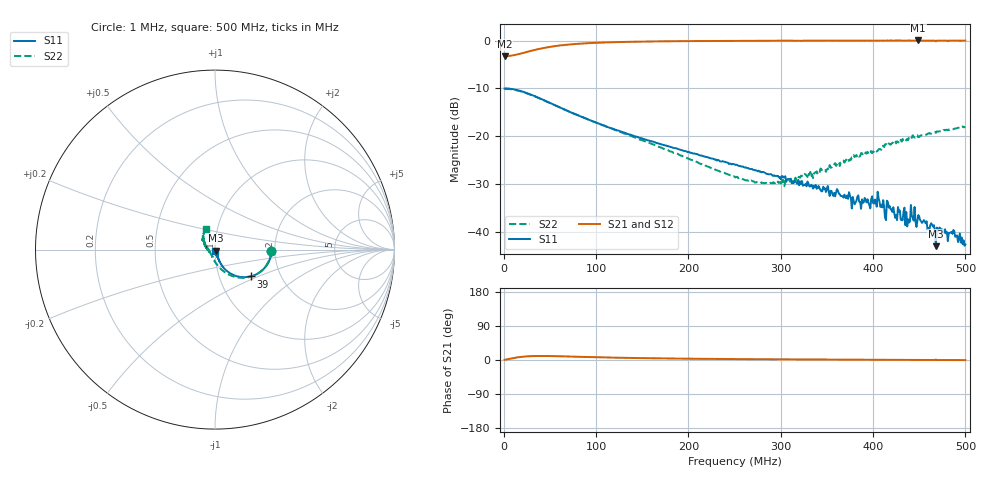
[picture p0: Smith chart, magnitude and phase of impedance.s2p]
# Hz S RI R 50.0
! written by SimSmith version 18.3b
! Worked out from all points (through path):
!   500 points, 1 MHz to 500 MHz, reference 50 ohm
!   highest |S21| = 0.01 dB at 449 MHz (marker M1); lowest = -3.3 dB at 1 MHz (marker M2)
!   group delay of S21, straight-line fit = 55.7 ps
!   lowest |S11| = -43.1 dB at 468 MHz (marker M3), VSWR 1.01, Z = 50.3 - j0.617 ohm
!   |S11| at or under -10 dB: start of sweep to end of sweep
!   |S22| runs from -30.5 to -10.1 dB; largest |S21 - S12| = 0
!   S11 on the Smith chart (normalised r, x): 1 MHz: 1.92, -0.03; 39 MHz: 1.41, -0.45; 500 MHz: 1.00, -0.01
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1000000  0.3147 -0.00637  0.6843 0.00685  0.6843 0.00685  0.3116 -0.00661
3.9e7  0.1984 -0.1495  0.8045 0.1515  0.8045 0.1515  0.1944 -0.1525
8.5e7  0.0853 -0.133  0.9203 0.1329  0.9203 0.1329  0.076 -0.1389
1.68e8  0.0313 -0.0774  0.9759 0.0738  0.9759 0.0738  0.00619 -0.0768
2.51e8  0.017 -0.0467  0.9899 0.0425  0.9899 0.0425  -0.0186 -0.0318
2.92e8  0.0124 -0.0362  0.9923 0.0315  0.9923 0.0315  -0.029 -0.0154
3.34e8  0.00921 -0.029  0.9952 0.0243  0.9952 0.0243  -0.0397 0.00337
3.74e8  0.00932 -0.0241  0.9973 0.0153  0.9973 0.0153  -0.051 0.0204
3.79e8  0.00652 -0.0199  0.9977 0.0154  0.9977 0.0154  -0.0581 0.0245
4.04e8  0.00586 -0.0172  0.997 0.0117  0.997 0.0117  -0.0596 0.0347
4.12e8  0.00624 -0.017  0.999 0.00941  0.999 0.00941  -0.0611 0.0465
4.17e8  0.00447 -0.0172  0.9976 0.00741  0.9976 0.00741  -0.0659 0.0512
4.24e8  0.00721 -0.0119  0.9986 0.00751  0.9986 0.00751  -0.0657 0.0587
4.34e8  0.00401 -0.0174  0.9961 0.00456  0.9961 0.00456  -0.0678 0.0631
4.37e8  0.00339 -0.0108  0.9979 0.00663  0.9979 0.00663  -0.0666 0.0656
4.43e8  0.00753 -0.0118  0.9988 0.00263  0.9988 0.00263  -0.0677 0.0761
4.49e8  0.00589 -0.0137  1.001 0.00264  1.001 0.00264  -0.0643 0.073
4.64e8  0.00272 -0.0114  0.9965 0.000988  0.9965 0.000988  -0.0635 0.0869
4.68e8  0.00345 -0.00613  0.9783 0.0228  0.9783 0.0228  -0.0631 0.0876
4.71e8  0.00223 -0.0104  0.9975 -0.000783  0.9975 -0.000783  -0.0624 0.0926
4.86e8  0.00289 -0.009  0.9971 -0.00137  0.9971 -0.00137  -0.0572 0.103
5e8  0.0012 -0.00722  0.998 -0.00419  0.998 -0.00419  -0.0497 0.1148
